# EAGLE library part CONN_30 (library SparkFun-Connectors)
Multi connection point. Often used as Generic Header-pin footprint for 0.1 inch spaced/style header connections On any of the 0.1 inch spaced packages, you can populate with these: Break Away Headers - Straight (PRT-00116) Break Away Male Headers - Right Angle (PRT-00553) Female Headers (PRT-00115) Break Away Headers - Machine Pin (PRT-00117) Break Away Female Headers - Swiss Machine Pin (PRT-00743) For SCREWTERMINALS and SPRING TERMINALS visit here: Screw Terimnals on SparkFun.com (5mm/3.5mm/2.54mm spacing) This device is also useful as a general connection point to wire up your design to another part of your project. Our various solder wires solder well into these plated through hole pads. Hook-Up Wire - Assortment (Stranded, 22 AWG) (PRT-11375) Hook-Up Wire - Assortment (Solid Core, 22 AWG) (PRT-11367) View the entire wire category on our website here Special notes: Molex polarized connector foot print use with SKU : PRT-08231 with associated crimp pins and housings. 1MM SMD Version SKU: PRT-10208 NOTES ON THE VARIANTS LOCK and LOCK_LONGPADS... This footprint was designed to help hold the alignment of a through-hole component (i.e. 6-pin header) while soldering it into place. You may notice that each hole has been shifted either up or down by 0.005 of an inch from it's more standard position (which is a perfectly straight line). This slight alteration caused the pins (the squares in the middle) to touch the edges of the holes. Because they are alternating, it causes a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
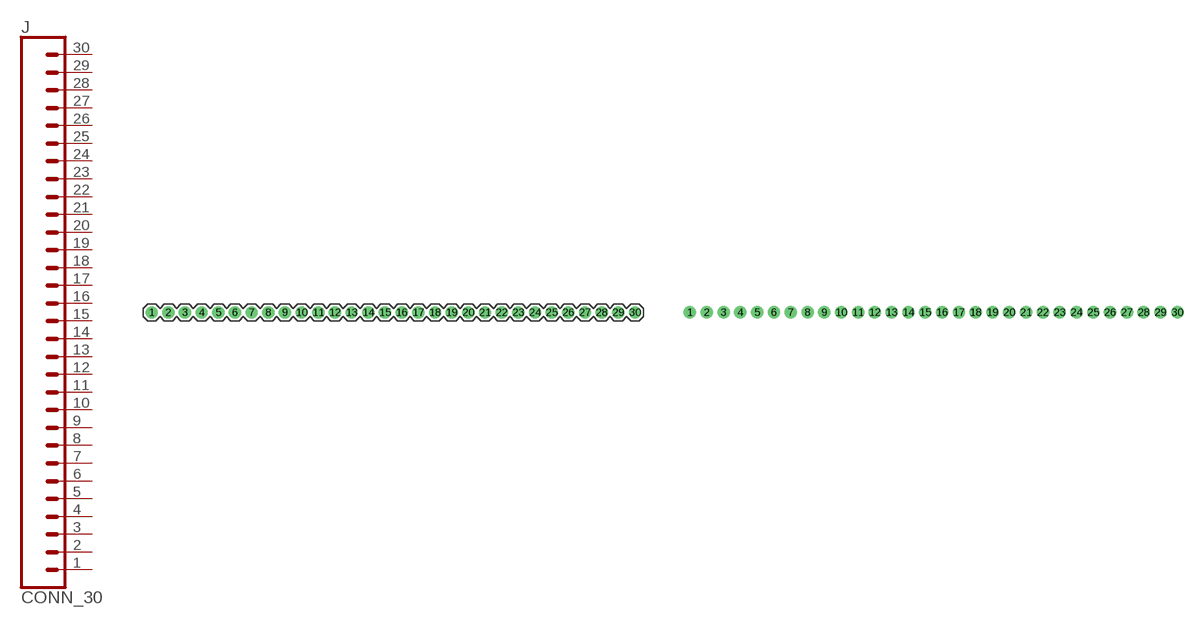
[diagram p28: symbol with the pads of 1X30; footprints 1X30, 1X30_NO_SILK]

Designator prefix J

## CONN_30  [1X30]
1  1  pas
2  2  pas
3  3  pas
4  4  pas
5  5  pas
6  6  pas
7  7  pas
8  8  pas
9  9  pas
10  10  pas
11  11  pas
12  12  pas
13  13  pas
14  14  pas
15  15  pas
16  16  pas
17  17  pas
18  18  pas
19  19  pas
20  20  pas
21  21  pas
22  22  pas
23  23  pas
24  24  pas
25  25  pas
26  26  pas
27  27  pas
28  28  pas
29  29  pas
30  30  pas

## CONN_30NO_SILK  [1X30_NO_SILK]
Pads as for 1X30

## Footprint 1X30 (pad centres in mm)
Plated Through Hole -30 Pins Specifications: Pin count:30 Pin pitch:0.1" Example device(s): CONN_30
drill 1.016 pad 1.88: 1 0,0; 2 2.54,0; 3 5.08,0; 4 7.62,0; 5 10.16,0; 6 12.7,0; 7 15.24,0; 8 17.78,0; 9 20.32,0; 10 22.86,0; 11 25.4,0; 12 27.94,0; 13 30.48,0; 14 33.02,0; 15 35.56,0; 16 38.1,0; 17 40.64,0; 18 43.18,0; 19 45.72,0; 20 48.26,0; 21 50.8,0; 22 53.34,0; 23 55.88,0; 24 58.42,0; 25 60.96,0; 26 63.5,0; 27 66.04,0; 28 68.58,0; 29 71.12,0; 30 73.66,0

## Footprint 1X30_NO_SILK (pad centres in mm)
Plated Through Hole -30 Pins No Silk Outline Specifications: Pin count:30 Pin pitch:0.1" Example device(s): CONN_30
drill 1.016 pad 1.88: 1 0,0; 2 2.54,0; 3 5.08,0; 4 7.62,0; 5 10.16,0; 6 12.7,0; 7 15.24,0; 8 17.78,0; 9 20.32,0; 10 22.86,0; 11 25.4,0; 12 27.94,0; 13 30.48,0; 14 33.02,0; 15 35.56,0; 16 38.1,0; 17 40.64,0; 18 43.18,0; 19 45.72,0; 20 48.26,0; 21 50.8,0; 22 53.34,0; 23 55.88,0; 24 58.42,0; 25 60.96,0; 26 63.5,0; 27 66.04,0; 28 68.58,0; 29 71.12,0; 30 73.66,0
